(* Logix 5000 DataType export InternalFlags; software revision 30.00 *)

TYPE InternalFlags :
STRUCT
   KsPrimeRequest : BOOL;
   CreateNewKsPrimeRequest : BOOL;
   KsIDMatchesMe : BOOL;
   KsPrimeIDMatchesMe : BOOL;
   MyPriDH : STRING;
   MyPubDH : STRING;
   PartnerLastPubDH : STRING;
   Ke : STRING;
END_STRUCT
END_TYPE
